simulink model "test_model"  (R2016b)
settings: Solver=VariableStepAuto  StartTime=0.0  StopTime=runtime  RelTol=1e-3
InitFcn:
  | clear mex
  | delete test_model_sfun.mexw64
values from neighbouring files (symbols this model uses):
  g = 9.81    [modelParameters.m]    (also in analyzeIMU_data.m = 9.8; getMomentOfInertia.m = 9.80665)
  height_controlled_o = (((Rm*If +      + (((omega0_o * 2 * Rm * Kv * Kq       * Kd + 1)^2) - 1)/(4* Rm*Kv^2*Kq      *Kd))/Vb)*(Pmax- Pmin)+Pmin)    [modelParameters.m]
  If = 0.511    [modelParameters.m]    (also in thrustDragConstantCalculations.m = [If0; If1; If2; If3]; Kd_error.m = I_0 * sign(rotor_speed_0) + I_1 * rotor_speed_0 + I_2 * roto)
  Jreq = 4.2012e-05    [modelParameters.m]
  Jxx = 0.0130    (= 0.013)    [modelParameters.m]
  Jyy = 0.0140    (= 0.014)    [modelParameters.m]
  Jzz = 0.0285    [modelParameters.m]
  Kd = 1.0317e-7    (= 1.0317e-07)    [modelParameters.m]    (also in calcDragConstant.m = ((A'*A)^-1)*A'*b; thrustDragConstantCalculations.m = calcDragConstant(data, Pmin, Pmax, Rm, Kv, Kq, If); Kd_error.m)
  Kq = 96.3422    [modelParameters.m]    (also in thrustDragConstantCalculations.m; Kd_error.m)
  Kt = 8.6519e-6    (= 8.6519e-06)    [modelParameters.m]    (also in calcThrustConstant.m = ((A'*A)^(-1))*(A'*T); thrustDragConstantCalculations.m = calcThrustConstant(data))
  Kv = 96.3422    [modelParameters.m]    (also in thrustDragConstantCalculations.m; Kd_error.m)
  m = 1.244    [modelParameters.m]
  omega0_o = (-1 + sqrt(1 - 4*Rm*Kv*Kq*Kd*( Kv*Rm*If - Kv*Vb_eff_0))) / (2*Rm*Kv*Kq*Kd)    [modelParameters.m]
  omega1_o = (-1 + sqrt(1 - 4*Rm*Kv*Kq*Kd*( Kv*Rm*If - Kv*Vb_eff_1))) / (2*Rm*Kv*Kq*Kd)    [modelParameters.m]
  omega2_o = (-1 + sqrt(1 - 4*Rm*Kv*Kq*Kd*( Kv*Rm*If - Kv*Vb_eff_2))) / (2*Rm*Kv*Kq*Kd)    [modelParameters.m]
  omega3_o = (-1 + sqrt(1 - 4*Rm*Kv*Kq*Kd*( Kv*Rm*If - Kv*Vb_eff_3))) / (2*Rm*Kv*Kq*Kd)    [modelParameters.m]
  pitch_o = pitch_value(1)    [modelParameters.m]
  pitchrate_o = pitchrate_value(1)    [modelParameters.m]
  Pmax = 2e5    (= 200000)    [modelParameters.m]    (also in thrustDragConstantCalculations.m; Kd_error.m)
  Pmin = 1e5    (= 100000)    [modelParameters.m]    (also in thrustDragConstantCalculations.m; Kd_error.m)
  rhx = 0.16    [modelParameters.m]
  rhy = 0.16    [modelParameters.m]
  rhz = 0.03    [modelParameters.m]
  Rm = 0.2308    [modelParameters.m]    (also in thrustDragConstantCalculations.m; Kd_error.m)
  roll_o = roll_value(1)    [modelParameters.m]
  rollrate_o = rollrate_value(1)    [modelParameters.m]
  Tc = 0.04    [modelParameters.m]
  Tq = 0.005    [modelParameters.m]
  Vb = 11.1    [modelParameters.m]    (also in calcDragConstant.m = [data.(6); data.(6); data.(6); data.(6)]; Kd_error.m = data.(6))
  x_controlled_o = 0    [modelParameters.m]
  x_o = x_position(1)    [modelParameters.m]
  x_vel_o = (x_position(2) - x_position(1)) / (time(2) - time(1))    [modelParameters.m]
  y_controlled_o = 0    [modelParameters.m]
  y_o = y_position(1)    [modelParameters.m]
  y_vel_o = (y_position(2) - y_position(1)) / (time(2) - time(1))    [modelParameters.m]
  yaw_controlled_o = 0    [modelParameters.m]
  yaw_o = yaw_value(1)    [modelParameters.m]
  yawrate_o = yawrate_value(1)    [modelParameters.m]
  z_o = z_position(1)    [modelParameters.m]
  z_vel_o = (z_position(2) - z_position(1)) / (time(2) - time(1))    [modelParameters.m]
undefined symbols (not defined in the file or in its folder): DiscIntNeverNeededParam
libraries: simulink x22, vrlib x2
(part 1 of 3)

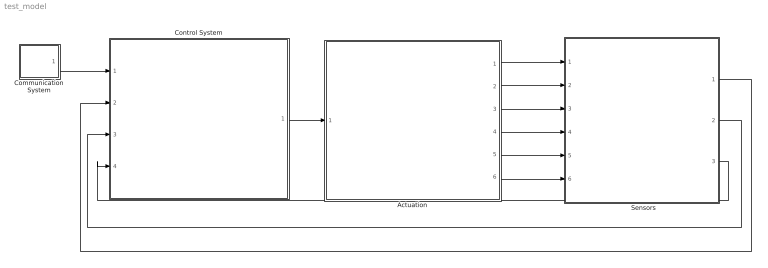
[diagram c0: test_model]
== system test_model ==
  "     Sensors   " : Subsystem
  Actuation : Subsystem
  Communication System : Subsystem
  Control System : Subsystem
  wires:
  Control System/1(P) -> Actuation/1(P)
  Communication System/1(setpoints) -> Control System/1(setpoints)
  Actuation/1(B_omega) -> "     Sensors   "/1(B_Omega)
  Actuation/2(euler_angles) -> "     Sensors   "/2(euler_angles)
  Actuation/3(B_vo) -> "     Sensors   "/3(B_vo)
  Actuation/4(E_ro) -> "     Sensors   "/4(E_ro)
  Actuation/5(B_vo_dot) -> "     Sensors   "/5(B_vo_dot)
  Actuation/6(B_g) -> "     Sensors   "/6(B_g)
  "     Sensors   "/3(current_position) -> Control System/4(current_position)
  "     Sensors   "/2(euler_rates) -> Control System/3(euler_rates)
  "     Sensors   "/1(euler_angles_filtered) -> Control System/2(euler_angles_filtered)

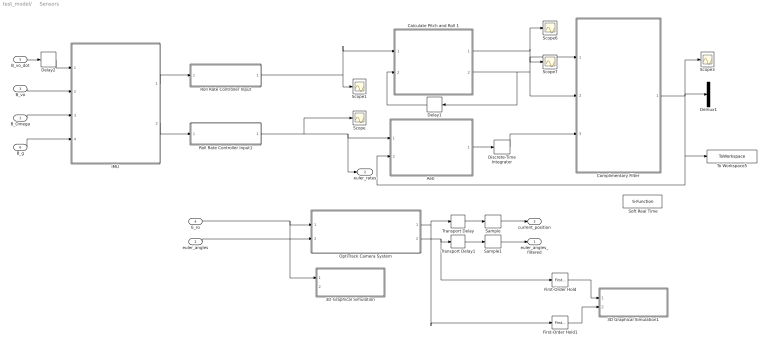
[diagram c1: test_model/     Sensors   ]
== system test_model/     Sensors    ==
  B_Omega : Inport
  euler_angles : Inport  Port=2
  B_vo : Inport  Port=3
  E_ro : Inport  Port=4
  B_vo_dot : Inport  Port=5
  B_g : Inport  Port=6
  3D Graphical Simulation : Subsystem  Commented=on
  3D Graphical Simulation1 : Subsystem  Commented=on
  "Aeb " : MATLAB Function  TreatAsAtomicUnit=on
  Calculate Pitch and Roll 1 : MATLAB Function  TreatAsAtomicUnit=on
  "Complimentary Filter " : MATLAB Function  TreatAsAtomicUnit=on
  Delay1 : Delay  DelayLength=1  InitialCondition=0  SampleTime=Tq
  Delay2 : Delay  DelayLength=1  InitialCondition=0  SampleTime=Tq
  Demux1 : Demux  Outputs=2
  Discrete-Time Integrator : DiscreteIntegrator  InitialConditionSetting=State (most efficient)  SampleTime=Tq  ICPrevOutput=DiscIntNeverNeededParam  ICPrevScaledInput=DiscIntNeverNeededParam
  First-Order Hold : simulink/Discrete/First-Order Hold  DisableCoverage=on  Ts=5e-3
  First-Order Hold1 : simulink/Discrete/First-Order Hold  DisableCoverage=on  Ts=5e-3
  "IMU " : Subsystem
  "OptiTrack Camera System " : Subsystem
  Roll Rate Controller Input : Subsystem  Variant=on
  Roll Rate Controller Input1 : Subsystem  Variant=on
  Sample : ZeroOrderHold  SampleTime=Tc
  Sample1 : ZeroOrderHold  SampleTime=Tc
  Scope{,1,3,6..7} (5 alike) : Scope
  Soft Real Time : S-Function  Commented=on  FunctionName=sfun_time  Parameters=x  SFunctionDeploymentMode=off  EnableBusSupport=off
  To Workspace5 : ToWorkspace  VariableName=angle_IMU_reading  SaveFormat=Structure With Time  SampleTime=Tq
  Transport Delay : TransportDelay  DelayTime=6e-3
  Transport Delay1 : TransportDelay  DelayTime=6e-3
  euler_angles_filtered : Outport
  euler_rates : Outport  Port=2
  current_position : Outport  Port=3
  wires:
  "IMU "/1(accelerometer) -> Roll Rate Controller Input/1(raw_accel_model)
  "IMU "/2(gyroscope) -> Roll Rate Controller Input1/1(raw_gyro_model)
  B_vo/1 -> "IMU "/2(B_vo)
  B_Omega/1 -> "IMU "/3(B_Omega)
  B_g/1 -> "IMU "/4(B_g)
  Calculate Pitch and Roll 1/2(accel_roll) -> Scope7/1, "Complimentary Filter "/2(accel_roll), Delay1/1
  Calculate Pitch and Roll 1/1(accel_pitch) -> Scope6/1, "Complimentary Filter "/1(accel_pitch)
  Delay1/1 -> Calculate Pitch and Roll 1/2(accel_roll_prev)
  euler_angles/1 -> "OptiTrack Camera System "/2(yaw)
  First-Order Hold/1 -> 3D Graphical Simulation1/1("Euler Angles ")
  E_ro/1 -> 3D Graphical Simulation/1(Displacement), "OptiTrack Camera System "/1(E_ro)
  First-Order Hold1/1 -> 3D Graphical Simulation1/2(Displacement)
  B_vo_dot/1 -> Delay2/1
  Delay2/1 -> "IMU "/1(B_vo_dot)
  "Aeb "/1(euler_rates_IMU) -> Discrete-Time Integrator/1
  Discrete-Time Integrator/1 -> "Complimentary Filter "/3(euler_angles_gyro)
  "OptiTrack Camera System "/1(E_ro_camera) -> Transport Delay/1, First-Order Hold1/1
  "OptiTrack Camera System "/2(yaw_camera) -> First-Order Hold/1, Transport Delay1/1
  Transport Delay/1 -> Sample/1
  Transport Delay1/1 -> Sample1/1
  Sample/1 -> current_position/1
  Sample1/1 -> euler_angles_filtered/1
  "Complimentary Filter "/1(euler_angles_IMU) -> To Workspace5/1, "Aeb "/2(euler_angles_IMU), Scope3/1, Demux1/1
  Roll Rate Controller Input/1(raw_accel) -> Scope1/1, Calculate Pitch and Roll 1/1(accel_reading)
  Roll Rate Controller Input1/1(raw_gyro) -> Scope/1, euler_rates/1, "Aeb "/1(gyro_reading)

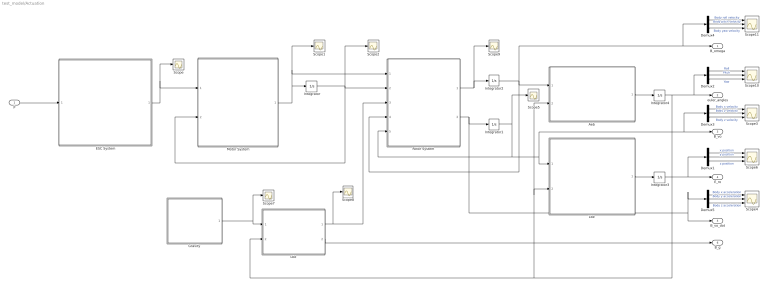
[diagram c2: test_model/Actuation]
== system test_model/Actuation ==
  P : Inport
  "Aeb " : MATLAB Function  TreatAsAtomicUnit=on
  Demux{1..5} (5 alike) : Demux  Outputs=3
  ESC System : MATLAB Function  TreatAsAtomicUnit=on
  "Gravity " : MATLAB Function  TreatAsAtomicUnit=on
  Integrator : Integrator  InitialCondition=[omega0_o, omega1_o, omega2_o, omega3_o]
  Integrator1 : Integrator  InitialCondition=[x_vel_o; y_vel_o; z_vel_o]
  Integrator2 : Integrator  InitialCondition=[rollrate_o; pitchrate_o; yawrate_o]
  Integrator3 : Integrator  InitialCondition=[x_o; y_o; z_o]
  Integrator4 : Integrator  InitialCondition=[roll_o; pitch_o; yaw_o]  ContinuousStateAttributes=['phi' 'theta' 'psi']
  "Lbe " : MATLAB Function  TreatAsAtomicUnit=on
  "Lbe " : MATLAB Function  TreatAsAtomicUnit=on
  Motor System : MATLAB Function  TreatAsAtomicUnit=on
  "Rotor System " : MATLAB Function  TreatAsAtomicUnit=on
  Scope{,1..2,5,7..9} (7 alike) : Scope
  Scope{3..4,6,10..11} (5 alike) : Scope  NumInputPorts=3
  B_omega : Outport
  euler_angles : Outport  Port=2
  B_vo : Outport  Port=3
  E_ro : Outport  Port=4
  B_vo_dot : Outport  Port=5
  B_g : Outport  Port=6
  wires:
  ESC System/1(Vb_eff) -> Scope/1, Motor System/1(Vb_eff)
  Motor System/1(w_dot) -> Integrator/1, "Rotor System "/1(w_dot), Scope1/1
  "Rotor System "/1(B_omega_dot) -> Scope9/1, Integrator2/1
  Integrator2/1 -> "Rotor System "/4(B_omega), B_omega/1, Demux4/1, "Aeb "/1(B_omega)
  "Aeb "/1(euler_rates) -> Integrator4/1
  "Lbe "/1(E_ro) -> Integrator3/1
  Integrator3/1 -> Demux1/1, E_ro/1
  "Lbe "/1(B_Fg) -> Scope8/1, "Rotor System "/3(B_Fg)
  "Lbe "/2(B_g) -> B_g/1
  Demux1/2 -> Scope6/2  "y position"
  Demux1/1 -> Scope6/1  "x position"
  Demux1/3 -> Scope6/3  "z position"
  Demux2/2 -> Scope10/2  "Pitch"
  Demux2/1 -> Scope10/1  "Roll"
  Demux2/3 -> Scope10/3  "Yaw"
  Demux4/2 -> Scope11/2  "Body pitch velocity"
  Demux4/1 -> Scope11/1  "Body roll velocity"
  Demux4/3 -> Scope11/3  "Body yaw velocity"
  Demux3/2 -> Scope3/2  "Body y velocity"
  Demux3/1 -> Scope3/1  "Body x velocity"
  Demux3/3 -> Scope3/3  "Body z velocity"
  Demux5/2 -> Scope4/2  "Body y acceleration"
  Demux5/1 -> Scope4/1  "Body x acceleration"
  Demux5/3 -> Scope4/3  "Body z acceleration"
  Integrator1/1 -> Scope5/1, "Rotor System "/5(B_vo), "Lbe "/1(B_vo), Demux3/1, B_vo/1
  "Rotor System "/2(B_vo_dot) -> Demux5/1, B_vo_dot/1, Integrator1/1
  Integrator4/1 -> euler_angles/1, Demux2/1, "Lbe "/2(euler_angles), "Aeb "/2(euler_angles), "Lbe "/2(euler_angles)
  P/1 -> ESC System/1(P)
  "Gravity "/1(E_Fg) -> Scope7/1, "Lbe "/1(E_Fg)
  Integrator/1 -> Motor System/2(w), "Rotor System "/2(w), Scope2/1

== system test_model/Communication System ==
  Step : Step  Before=[0; 0; 0; 0]  After=[1; 1; 0; 0]  SampleTime=Tq
  setpoints : Outport
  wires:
  Step/1 -> setpoints/1

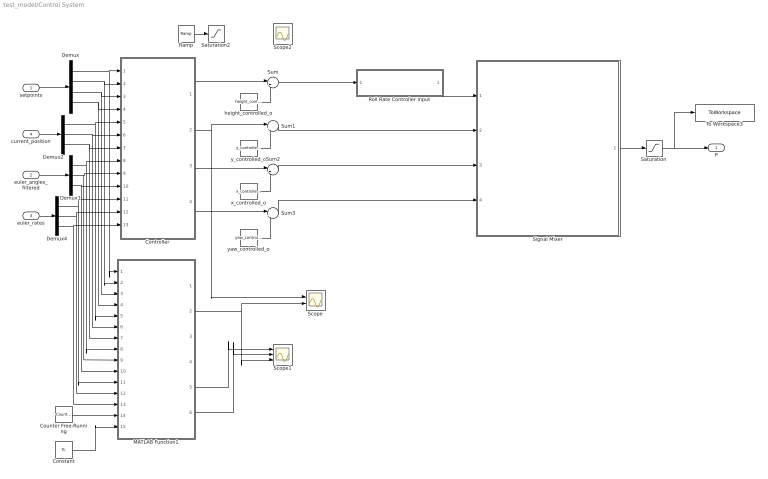
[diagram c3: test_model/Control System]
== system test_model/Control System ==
  setpoints : Inport
  euler_angles_filtered : Inport  Port=2
  euler_rates : Inport  Port=3
  current_position : Inport  Port=4
  Constant : Constant  Value=Tc  SampleTime=Tc
  Controller : Subsystem
  Counter Free-Running : simulink/Sources/Counter Free-Running  NumBits=32  tsamp=Tc
  Demux : Demux
  Demux1 : Demux  Outputs=3
  Demux2 : Demux  Outputs=3
  Demux4 : Demux  Outputs=3
  MATLAB Function1 : MATLAB Function  TreatAsAtomicUnit=on  SystemSampleTime=Tq
  Ramp : simulink/Sources/Ramp  slope=2*height_controlled_o  start=6.32  X0=0
  Roll Rate Controller Input : Subsystem  Variant=on
  Saturation : Saturate  UpperLimit=Pmax*ones(4,1)  LowerLimit=Pmin*ones(4,1)
  Saturation2 : Saturate  UpperLimit=height_controlled_o  LowerLimit=0
  Scope : Scope  NumInputPorts=2
  Scope1 : Scope  NumInputPorts=3
  Scope2 : Scope
  Signal Mixer : MATLAB Function  TreatAsAtomicUnit=on
  Sum{,1..3} (4 alike) : Sum  Inputs=|++
  To Workspace3 : ToWorkspace  VariableName=motorCommands  SaveFormat=Structure With Time  SampleTime=Tq
  height_controlled_o : Constant  Value=height_controlled_o  SampleTime=Tc
  x_controlled_o : Constant  Value=x_controlled_o
  y_controlled_o : Constant  Value=y_controlled_o
  yaw_controlled_o : Constant  Value=yaw_controlled_o
  P : Outport
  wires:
  setpoints/1 -> Demux/1
  euler_angles_filtered/1 -> Demux1/1
  current_position/1 -> Demux2/1
  euler_rates/1 -> Demux4/1
  Demux/1 -> MATLAB Function1/1(set_x), Controller/1(x_setpoint)
  Demux/2 -> MATLAB Function1/2(set_y), Controller/2(y_setpoint)
  Demux/3 -> MATLAB Function1/3(set_z), Controller/3(z_setpoint)
  Demux2/1 -> MATLAB Function1/5(cur_x), Controller/5(x_position)
  Demux2/2 -> Controller/6(y_position), MATLAB Function1/6(cur_y)
  Demux2/3 -> MATLAB Function1/7(cur_z), Controller/7(z_position)
  Controller/2(y_controlled) -> Scope/1, Sum1/1
  Controller/4(yaw_controlled) -> Sum3/1
  y_controlled_o/1 -> Sum1/2
  x_controlled_o/1 -> Sum2/2
  yaw_controlled_o/1 -> Sum3/2
  Signal Mixer/1(P) -> Saturation/1
  Demux1/1 -> Controller/8(roll), MATLAB Function1/8(cur_phi)
  Demux1/2 -> MATLAB Function1/9(cur_theta), Controller/9(pitch)
  Demux4/1 -> Controller/11(roll_rate), MATLAB Function1/11(cur_phi_d)
  Demux4/2 -> Controller/12(pitch_rate), MATLAB Function1/12(cur_theta_d)
  Demux4/3 -> MATLAB Function1/13(cur_psi_d), Controller/13(yaw_rate)
  Demux/4 -> MATLAB Function1/4(set_yaw), Controller/4(yaw_setpoint)
  Demux1/3 -> MATLAB Function1/10(cur_psi), Controller/10(yaw)
  Controller/3(x_controlled) -> Sum2/1
  Counter Free-Running/1 -> MATLAB Function1/14(vrpn_id)
  Constant/1 -> MATLAB Function1/15(Tc)
  Sum/1 -> Roll Rate Controller Input/1(z_command_model)
  MATLAB Function1/5(pid_y_out) -> Scope1/1
  MATLAB Function1/6(pid_roll_out) -> Scope1/2
  MATLAB Function1/2(y_cor) -> Scope1/3, Scope/2
  Ramp/1 -> Saturation2/1
  height_controlled_o/1 -> Sum/2
  Saturation/1 -> To Workspace3/1, P/1
  Controller/1(height_controlled) -> Sum/1
  Roll Rate Controller Input/1(z_command) -> Signal Mixer/1(height_controlled)
  Sum1/1 -> Signal Mixer/2(y_controlled)
  Sum2/1 -> Signal Mixer/3(x_controlled)
  Sum3/1 -> Signal Mixer/4(yaw_controlled)

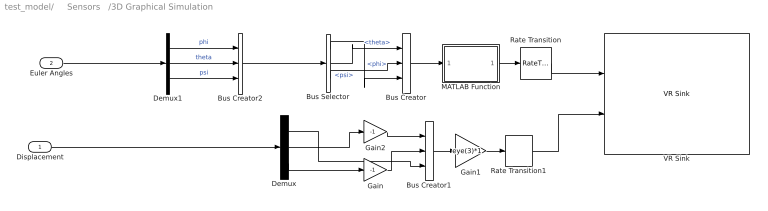
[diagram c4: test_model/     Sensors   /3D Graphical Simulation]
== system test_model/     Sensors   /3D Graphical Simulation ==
  Displacement : Inport
  Euler Angles : Inport  Port=2
  Bus Creator : BusCreator  Inputs=3
  Bus Creator1 : BusCreator  Inputs=3
  Bus Creator2 : BusCreator  Inputs=3
  Bus Selector : BusSelector  OutputSignals=phi,theta,psi
  Demux : Demux  Outputs=3
  Demux1 : Demux  Outputs=3
  Gain : Gain  Gain=-1
  Gain1 : Gain  Gain=eye(3)*1  Multiplication=Matrix(K*u)
  Gain2 : Gain  Gain=-1
  MATLAB Function : MATLAB Function  TreatAsAtomicUnit=on
  Rate Transition : RateTransition  OutPortSampleTime=0.06
  Rate Transition1 : RateTransition  OutPortSampleTime=0.06
  VR Sink : vrlib/VR Sink  InstantiateOnLoad=on  SampleTime=-1  ViewEnable=on  RemoteChange=off  RemoteView=off  FieldsWritten=Helicopter.rotation.4.1.1.double#Helicopter.translation.3.1.1.double  WorldFileName=quadrotor_world_ucart.wrl  AutoView=on  VideoDimensions=[]  AllowVariableSize=off
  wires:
  Displacement/1 -> Demux/1
  Bus Creator2/1 -> Bus Selector/1
  Demux/1 -> Bus Creator1/3
  Gain/1 -> Bus Creator1/2
  Gain2/1 -> Bus Creator1/1
  Rate Transition1/1 -> VR Sink/2
  Rate Transition/1 -> VR Sink/1
  Demux/3 -> Gain/1
  Demux/2 -> Gain2/1
  Bus Creator1/1 -> Gain1/1
  Bus Selector/1 -> Bus Creator/3  "<phi>"
  Bus Selector/3 -> Bus Creator/2  "<psi>"
  Bus Selector/2 -> Bus Creator/1  "<theta>"
  Gain1/1 -> Rate Transition1/1
  Demux1/3 -> Bus Creator2/3  "psi"
  Demux1/2 -> Bus Creator2/2  "theta"
  Demux1/1 -> Bus Creator2/1  "phi"
  Euler Angles/1 -> Demux1/1
  Bus Creator/1 -> MATLAB Function/1(u)
  MATLAB Function/1(y) -> Rate Transition/1

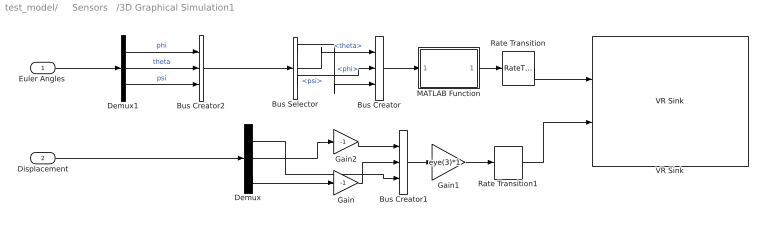
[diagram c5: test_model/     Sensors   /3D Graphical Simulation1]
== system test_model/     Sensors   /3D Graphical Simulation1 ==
  "Euler Angles " : Inport
  Displacement : Inport  Port=2
  Bus Creator : BusCreator  Inputs=3
  Bus Creator1 : BusCreator  Inputs=3
  Bus Creator2 : BusCreator  Inputs=3
  Bus Selector : BusSelector  OutputSignals=phi,theta,psi
  Demux : Demux  Outputs=3
  Demux1 : Demux  Outputs=3
  Gain : Gain  Gain=-1
  Gain1 : Gain  Gain=eye(3)*1  Multiplication=Matrix(K*u)
  Gain2 : Gain  Gain=-1
  MATLAB Function : MATLAB Function  TreatAsAtomicUnit=on
  Rate Transition : RateTransition  OutPortSampleTime=0.06
  Rate Transition1 : RateTransition  OutPortSampleTime=0.06
  VR Sink : vrlib/VR Sink  InstantiateOnLoad=on  SampleTime=-1  ViewEnable=on  RemoteChange=off  RemoteView=off  FieldsWritten=Helicopter.rotation.4.1.1.double#Helicopter.translation.3.1.1.double  WorldFileName=quadrotor_world_ucart.wrl  AutoView=on  VideoDimensions=[]  AllowVariableSize=off
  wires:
  Bus Creator2/1 -> Bus Selector/1
  Demux/1 -> Bus Creator1/3
  Gain/1 -> Bus Creator1/2
  Gain2/1 -> Bus Creator1/1
  Rate Transition1/1 -> VR Sink/2
  Rate Transition/1 -> VR Sink/1
  Demux/3 -> Gain/1
  Demux/2 -> Gain2/1
  Bus Creator1/1 -> Gain1/1
  Bus Selector/1 -> Bus Creator/3  "<phi>"
  Bus Selector/3 -> Bus Creator/2  "<psi>"
  Bus Selector/2 -> Bus Creator/1  "<theta>"
  Gain1/1 -> Rate Transition1/1
  Demux1/3 -> Bus Creator2/3  "psi"
  Demux1/2 -> Bus Creator2/2  "theta"
  Demux1/1 -> Bus Creator2/1  "phi"
  Bus Creator/1 -> MATLAB Function/1(u)
  MATLAB Function/1(y) -> Rate Transition/1
  Displacement/1 -> Demux/1
  "Euler Angles "/1 -> Demux1/1

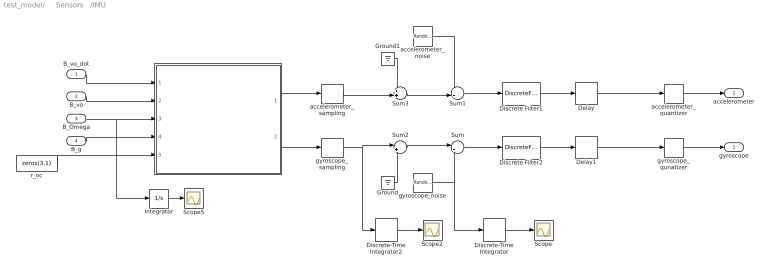
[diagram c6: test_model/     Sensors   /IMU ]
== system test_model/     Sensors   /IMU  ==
  B_vo_dot : Inport
  B_vo : Inport  Port=2
  B_Omega : Inport  Port=3
  B_g : Inport  Port=4
  " " : MATLAB Function  TreatAsAtomicUnit=on
  Delay : Delay  DelayLength=4  InitialCondition=0  SampleTime=Tq
  Delay1 : Delay  DelayLength=4  InitialCondition=0  SampleTime=Tq
  Discrete Filter1 : DiscreteFilter  Numerator=[0 0.1454]  Denominator=[1 -0.8546]  SampleTime=Tq
  Discrete Filter2 : DiscreteFilter  Numerator=[0 0.1454]  Denominator=[1 -0.8546]  SampleTime=Tq
  Discrete-Time Integrator : DiscreteIntegrator  InitialConditionSetting=State (most efficient)  SampleTime=-1  ICPrevOutput=DiscIntNeverNeededParam  ICPrevScaledInput=DiscIntNeverNeededParam
  Discrete-Time Integrator2 : DiscreteIntegrator  InitialConditionSetting=State (most efficient)  SampleTime=-1  ICPrevOutput=DiscIntNeverNeededParam  ICPrevScaledInput=DiscIntNeverNeededParam
  Ground : Ground
  Ground1 : Ground
  Integrator : Integrator
  Scope : Scope
  Scope2 : Scope
  Scope5 : Scope
  Sum : Sum  Inputs=|++
  Sum1 : Sum  Inputs=++|
  Sum2 : Sum  Inputs=|++
  Sum3 : Sum  Inputs=++|
  accelerometer_noise : RandomNumber  Mean=zeros(3,1)  Variance=[ 3e-7 ; 3.3e-7 ; 7.2e-7 ]  Seed=[0,1,2]  SampleTime=Tq
  accelerometer_quantizer : Quantizer  QuantizationInterval=2.4400e-04
  accelerometer_sampling : ZeroOrderHold  SampleTime=Tq
  gyroscope_noise : RandomNumber  Mean=zeros(3,1)  Variance=[ 2.2e-8 ; 1.1e-7 ; 2.4e-8 ]  Seed=[0,1,2]  SampleTime=Tq
  gyroscope_qunatizer : Quantizer  QuantizationInterval=1.1e-3
  gyroscope_sampling : ZeroOrderHold  SampleTime=Tq
  r_oc : Constant  Value=zeros(3,1)
  accelerometer : Outport
  gyroscope : Outport  Port=2
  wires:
  accelerometer_noise/1 -> Sum1/1
  Sum/1 -> Discrete Filter2/1
  Sum2/1 -> Sum/1
  Sum3/1 -> Sum1/2
  gyroscope_noise/1 -> Sum/2, Discrete-Time Integrator/1
  Sum1/1 -> Discrete Filter1/1
  gyroscope_sampling/1 -> Sum2/1, Discrete-Time Integrator2/1
  accelerometer_sampling/1 -> Sum3/2
  Ground/1 -> Sum2/2
  Ground1/1 -> Sum3/1
  B_vo_dot/1 -> " "/1(B_vo_dot)
  B_vo/1 -> " "/2(B_vo)
  B_Omega/1 -> Integrator/1, " "/3(B_Omega)
  B_g/1 -> " "/4(B_g)
  r_oc/1 -> " "/5(r_oc)
  " "/2(gyroReading) -> gyroscope_sampling/1
  " "/1(accelReading) -> accelerometer_sampling/1
  Discrete-Time Integrator/1 -> Scope/1
  Discrete-Time Integrator2/1 -> Scope2/1
  Integrator/1 -> Scope5/1
  gyroscope_qunatizer/1 -> gyroscope/1
  accelerometer_quantizer/1 -> accelerometer/1
  Discrete Filter2/1 -> Delay1/1
  Discrete Filter1/1 -> Delay/1
  Delay/1 -> accelerometer_quantizer/1
  Delay1/1 -> gyroscope_qunatizer/1

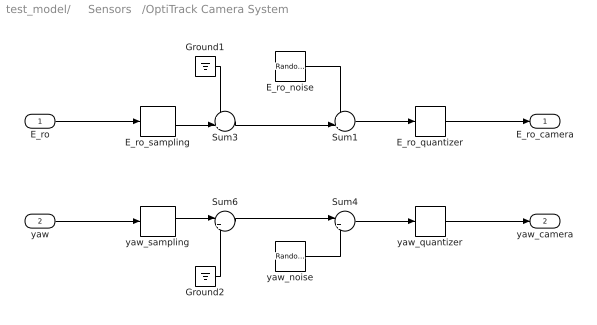
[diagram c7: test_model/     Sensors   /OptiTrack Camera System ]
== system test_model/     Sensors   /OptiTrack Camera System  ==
  E_ro : Inport
  yaw : Inport  Port=2
  E_ro_noise : RandomNumber  Mean=zeros(3,1)  Variance=[ 7.9664e-10 ; 1.1928e-10 ; 5.0636e-10 ]  Seed=[0,1,2]  SampleTime=Tc
  E_ro_quantizer : Quantizer  QuantizationInterval=2.4400e-04
  E_ro_sampling : ZeroOrderHold  SampleTime=Tc
  Ground1 : Ground
  Ground2 : Ground
  Sum1 : Sum  Inputs=++|
  Sum3 : Sum  Inputs=++|
  Sum4 : Sum  Inputs=|++
  Sum6 : Sum  Inputs=|++
  yaw_noise : RandomNumber  Variance=1.0783e-9  SampleTime=Tc
  yaw_quantizer : Quantizer  QuantizationInterval=1.1e-3
  yaw_sampling : ZeroOrderHold  SampleTime=Tc
  E_ro_camera : Outport
  yaw_camera : Outport  Port=2
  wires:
  E_ro_noise/1 -> Sum1/1
  Sum3/1 -> Sum1/2
  Sum1/1 -> E_ro_quantizer/1
  E_ro_sampling/1 -> Sum3/2
  Ground1/1 -> Sum3/1
  Sum4/1 -> yaw_quantizer/1
  Sum6/1 -> Sum4/1
  yaw_noise/1 -> Sum4/2
  yaw_sampling/1 -> Sum6/1
  Ground2/1 -> Sum6/2
  yaw/1 -> yaw_sampling/1
  E_ro/1 -> E_ro_sampling/1
  E_ro_quantizer/1 -> E_ro_camera/1
  yaw_quantizer/1 -> yaw_camera/1

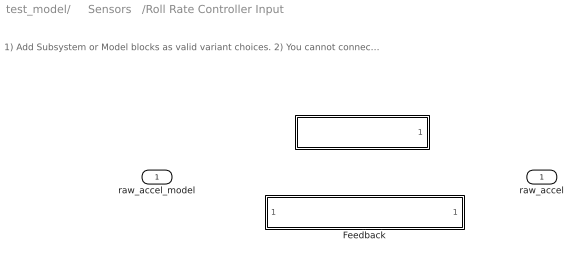
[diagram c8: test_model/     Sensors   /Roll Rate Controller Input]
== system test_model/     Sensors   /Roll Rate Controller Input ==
  note: 1) Add Subsystem or Model blocks as valid variant choices. 2) You cannot connect blocks at this level. At simulation, connectivity is automatically determined, based on the active variant and port name matching.
  raw_accel_model : Inport
  " " : Subsystem  VariantControl=logAnalysisToggle==1
  Feedback : Subsystem  VariantControl=logAnalysisToggle==0
  raw_accel : Outport

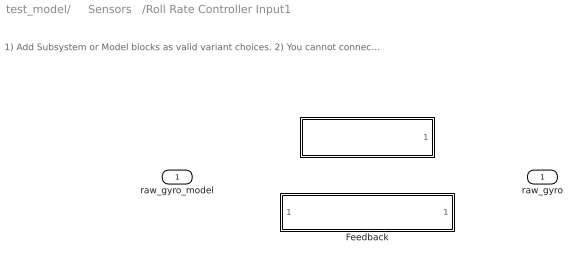
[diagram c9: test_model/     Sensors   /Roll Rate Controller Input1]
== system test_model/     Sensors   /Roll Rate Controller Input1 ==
  note: 1) Add Subsystem or Model blocks as valid variant choices. 2) You cannot connect blocks at this level. At simulation, connectivity is automatically determined, based on the active variant and port name matching.
  raw_gyro_model : Inport
  " " : Subsystem  VariantControl=logAnalysisToggle==1
  Feedback : Subsystem  VariantControl=logAnalysisToggle==0
  raw_gyro : Outport
